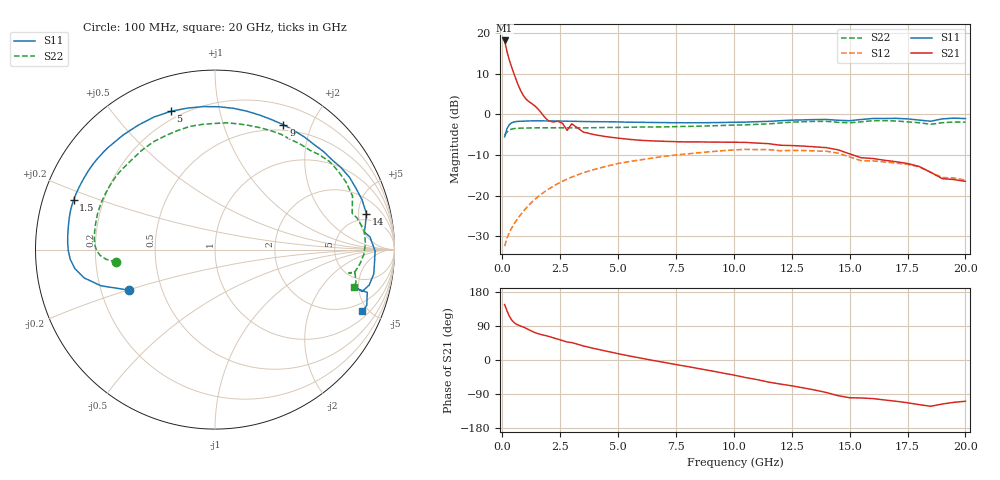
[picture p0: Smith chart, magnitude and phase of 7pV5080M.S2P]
! Infineon Technologies  Discrete & RF Semiconductors
! bfp620
! VCE = 0.50 V,  IC =  80 mA
! Common Emitter S-Parameters:  Sep 2002
# GHz  S  MA  R  50
!  f  S11  S21  S12  S22
! GHz  MAG  ANG  MAG  ANG  MAG  ANG  MAG  ANG
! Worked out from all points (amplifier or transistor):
!   59 points, 100 MHz to 20 GHz, reference 50 ohm
!   highest |S21| = 18.2 dB at 100 MHz (marker M1)
!   |S21| within 3 dB of that: start of sweep to 214.6 MHz
!   unconditionally stable (mu >= 1): start of sweep to end of sweep
!   at 1 GHz: K = 1.35, MAG = 10.1 dB, |S12| = -23.2 dB
!   at 5.5 GHz: K = 1.32, MAG = -0.7 dB, |S12| = -11.6 dB
!   at 20 GHz: K = 2.30, MAG = -6.6 dB, |S12| = -16.2 dB
!   S11 on the Smith chart (normalised r, x): 100 MHz: 0.32, -0.20; 1.5 GHz: 0.09, +0.17; 5 GHz: 0.16, +0.72; 9 GHz: 0.43, +1.60; 14 GHz: 3.86, +6.22; 20 GHz: 1.41, -4.59
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0.1  0.5286 -154.7  8.144 146.4  0.0239 26.4  0.554 -172.8
0.2  0.6668 -162.4  5.97 130.2  0.0298 32.7  0.6094 -174.9
0.3  0.746 -167.8  4.703 116.3  0.035 37.1  0.6417 -177.2
0.4  0.788 -172.3  3.851 106.1  0.0398 40.5  0.6597 -179.6
0.5  0.8085 -176.2  3.196 99.2  0.0444 43.2  0.6691 178.1
0.6  0.8177 -179.7  2.67 94.8  0.0491 45.4  0.6739 175.8
0.7  0.8218 177.2  2.256 91.9  0.0538 47.1  0.6763 173.7
0.9  0.8261 172.1  1.727 87.1  0.0637 49.3  0.679 170.0
1.5  0.8349 160.7  1.202 70.4  0.0948 49.9  0.6847 160.6
2  0.8317 151.6  0.835 62.4  0.1206 46.9  0.6854 153.0
2.4  0.8302 145.5  0.826 54.9  0.1408 43.5  0.6859 147.3
2.8  0.8255 138.9  0.637 47.5  0.1601 39.6  0.6855 141.5
3  0.8238 136.3  0.767 46.0  0.1695 37.5  0.6842 139.0
3.5  0.8182 128.6  0.607 37.1  0.1922 31.9  0.6826 132.4
5  0.8088 107.6  0.511 16.7  0.2489 15.4  0.692 113.3
7  0.7939 82.6  0.467 -6.4  0.3051 -6.0  0.7027 90.2
9  0.7932 61.3  0.457 -28.4  0.3479 -27.3  0.7241 69.8
10.5  0.8047 46.6  0.453 -46.2  0.3715 -45.3  0.7442 55.5
13.5  0.865 18.6  0.399 -79.3  0.356 -78.5  0.8212 27.2
14  0.8673 13.3  0.39 -85.9  0.3525 -85.3  0.8225 21.3
17  0.895 -8.7  0.262 -108.8  0.2518 -108.9  0.8299 -1.8
20  0.889 -22.6  0.15 -108.9  0.1554 -120.9  0.8037 -15.0
